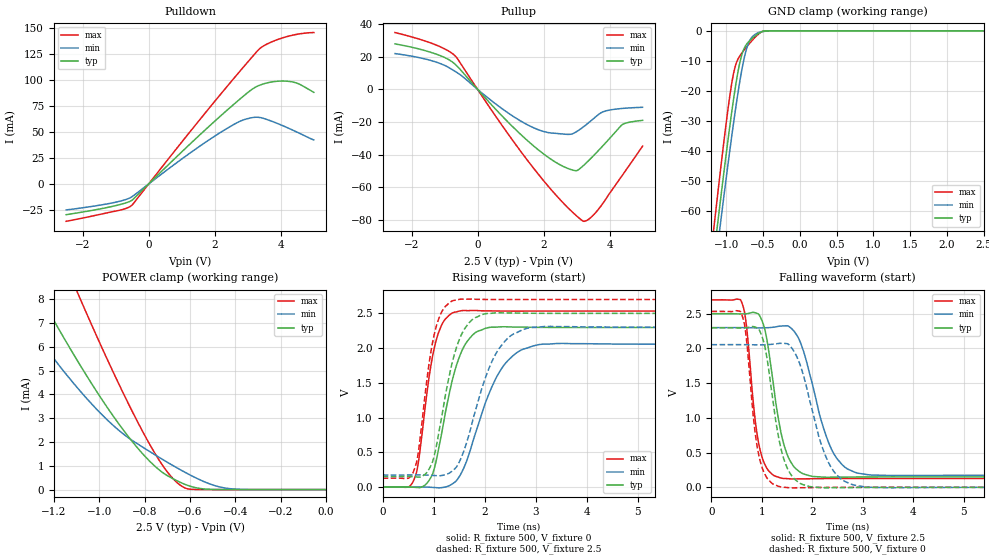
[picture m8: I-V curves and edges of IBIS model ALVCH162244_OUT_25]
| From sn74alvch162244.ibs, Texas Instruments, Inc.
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[Model]   ALVCH162244_OUT_25
Model_type  3-state
Enable   Active-Low
Vref =   0
Rref =   500
Cref =   30p
Vmeas =   1.25
| variable   typ   min   max
C_comp   7.01pF   5.81pF   8.07pF
| C_pullup   5.45pF   4.15pF   8.21pF
| C_pulldown   4.49pF   3.97pF   5.46pF
| C_tri-state   7.01pF   5.81pF   8.07pF
[Temperature Range]   40   100   -40
| Ambient temperature   25   85   -40
[Voltage range]   2.5   2.3   2.7
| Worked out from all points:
|   slope of the pulldown table from 0 to 0.375 V, typ, clamps not added: 32.2 ohm
|   slope of the pullup table from 0 to 0.375 V, typ, clamps not added: 44.6 ohm
|   GND clamp passes 1 mA (typ) near -0.57 V on its own axis
|   POWER clamp passes 1 mA (typ) near -0.76 V on its own axis
|   rising waveform, R_fixture 500, V_fixture 0: 20-80 % time 414ps typ, 616ps min, 291ps max; typ from 0 V to 2.3 V
|   falling waveform, R_fixture 500, V_fixture 2.5: 20-80 % time 313ps typ, 488ps min, 220ps max; typ from 2.5 V to 0.151 V
|   rising waveform, R_fixture 500, V_fixture 2.5: 20-80 % time 396ps typ, 559ps min, 284ps max; typ from 0.151 V to 2.5 V
|   falling waveform, R_fixture 500, V_fixture 0: 20-80 % time 307ps typ, 476ps min, 218ps max; typ from 2.3 V to 0 V
[GND Clamp]
| ALVCH162244_OUT_25
|   Voltage   I(typ)   I(min)   I(max)
-2.5V     -368.1mA   -367.2mA   -371.3mA
-1.175V   -76.67mA   -83.94mA   -67.56mA
-1.12V    -65.28mA   -72.86mA   -55.65mA
-1.075V   -56.11mA   -63.91mA   -46.11mA
-960mV    -33.67mA   -41.79mA   -23.46mA
-880mV    -19.7mA    -27.44mA   -12.2mA
-805mV    -9.656mA   -15.54mA   -8.049mA
-730mV    -4.751mA   -6.651mA   -5.626mA
-670mV    -3.059mA   -2.851mA   -3.862mA
-590mV    -1.419mA   -939uA     -1.764mA
-460mV    -11.33uA   -126uA     -6.688uA
2.5V      83.81pA    43.81nA    39.19pA
[POWER Clamp]
| ALVCH162244_OUT_25
|   Voltage   I(typ)   I(min)   I(max)
-2.5V     32.96mA    25.76mA    44.33mA
-1.415V   10.88mA    8.346mA    15.71mA
-1.39V    10.43mA    7.998mA    15.1mA
-1.265V   8.212mA    6.323mA    12.13mA
-1.095V   5.397mA    4.263mA    8.259mA
-1.075V   5.085mA    4.041mA    7.82mA
-945mV    3.18mA     2.753mA    5.07mA
-835mV    1.794mA    1.945mA    2.921mA
-725mV    748.5uA    1.292mA    1.078mA
-645mV    315uA      848.1uA    201uA
-430mV    586.9nA    45uA       19.76nA
-31.15fV  83.81pA    322.9pA    46.7pA
[Pulldown]
| ALVCH162244_OUT_25
|   Voltage   I(typ)   I(min)   I(max)
-2.5V     -29.57mA   -25mA      -35.92mA
-1.11V    -21.64mA   -18.3mA    -26.79mA
-720mV    -18.47mA   -15.27mA   -23.9mA
-510mV    -15.74mA   -12.3mA    -20.47mA
1.71V     51.84mA    39.79mA    68.05mA
2.535V    75.28mA    56.31mA    99.7mA
2.96V     86.7mA     62.36mA    115.6mA
3.205V    92.39mA    63.96mA    124.6mA
3.41V     95.38mA    63.53mA    131.1mA
4.02V     98.8mA     56.47mA    139.9mA
4.49V     96.76mA    49.79mA    143.7mA
5V        87.96mA    42.25mA    145.4mA
[Pullup]
| ALVCH162244_OUT_25
|   Voltage   I(typ)   I(min)   I(max)
-2.5V     27.76mA    21.84mA    34.68mA
-1.295V   21.81mA    16.89mA    27.4mA
-680mV    15.33mA    10.96mA    20.45mA
795mV     -17.39mA   -12.61mA   -23.59mA
1.72V     -35mA      -23.72mA   -48.83mA
2.725V    -48.31mA   -27.56mA   -72.15mA
2.995V    -49.8mA    -25.98mA   -77.31mA
3.195V    -46.88mA   -23.17mA   -80.61mA
3.595V    -38.91mA   -16.57mA   -75.04mA
3.855V    -33.31mA   -13.41mA   -68.1mA
4.37V     -21.83mA   -11.74mA   -53.08mA
5V        -19mA      -11.01mA   -34.76mA
[Ramp]
| ALVCH162244_OUT_25
| variable   typ   min   max
dV/dt_r   1.39/4.27E-10   1.25/6.48E-10   1.53/3.02E-10
dV/dt_f   1.42/3.31E-10   1.29/5.15E-10   1.55/2.30E-10
R_load = 500
[Rising Waveform]
| ALVCH162244_OUT_25
R_fixture =   500
C_fixture =   0
L_fixture =   0
V_fixture =   0
V_fixture_min = 0
V_fixture_max = 0
|   Time   V(typ)   V(min)   V(max)
0s        249.4uV    275uV      221.5uV
620ps     -2.589mV   2.187mV    116.2mV
710ps     -6.682mV   2.508mV    398.7mV
940ps     131.6mV    -2.695mV   1.72V
1.185ns   882.8mV    -4.875mV   2.372V
1.565ns   1.979V     233.7mV    2.541V
1.84ns    2.233V     818.6mV    2.541V
2.315ns   2.307V     1.686V     2.534V
3.155ns   2.299V     2.059V     2.533V
40ns      2.297V     2.055V     2.533V
[Falling Waveform]
| ALVCH162244_OUT_25
R_fixture =   500
C_fixture =   0
L_fixture =   0
V_fixture =   2.5
V_fixture_min = 2.3
V_fixture_max = 2.7
|   Time   V(typ)   V(min)   V(max)
0s        2.5V       2.3V       2.7V
620ps     2.497V     2.3V       2.625V
690ps     2.499V     2.299V     2.354V
960ps     2.466V     2.296V     553.9mV
1.095ns   2.147V     2.298V     279.6mV
1.435ns   620.9mV    2.325V     127mV
1.765ns   215.7mV    2.085V     122.4mV
2.435ns   146.8mV    474.3mV    126.6mV
3.165ns   149.6mV    177.1mV    127.2mV
40ns      150.8mV    173.8mV    127mV
[Rising Waveform]
| ALVCH162244_OUT_25
R_fixture =   500
C_fixture =   0
L_fixture =   0
V_fixture =   2.5
V_fixture_min = 2.3
V_fixture_max = 2.7
|   Time   V(typ)   V(min)   V(max)
0s        151mV      174.1mV    127.3mV
610ps     148.1mV    175.6mV    232.1mV
705ps     143.9mV    175.7mV    528.4mV
920ps     272.3mV    170.5mV    1.826V
1.165ns   1.039V     167.7mV    2.53V
1.355ns   1.764V     225.7mV    2.676V
1.535ns   2.178V     412.9mV    2.704V
2.255ns   2.509V     1.962V     2.7V
3.16ns    2.501V     2.311V     2.7V
40ns      2.5V       2.3V       2.7V
[Falling Waveform]
| ALVCH162244_OUT_25
R_fixture =   500
C_fixture =   0
L_fixture =   0
V_fixture =   0
V_fixture_min = 0
V_fixture_max = 0
|   Time   V(typ)   V(min)   V(max)
0s        2.297V     2.054V     2.533V
610ps     2.295V     2.055V     2.473V
685ps     2.297V     2.054V     2.194V
945ps     2.271V     2.052V     444mV
1.075ns   1.971V     2.054V     167.1mV
1.42ns    444.7mV    2.073V     375.5uV
1.73ns    71.1mV     1.821V     -5.64mV
2.375ns   -5.73mV    285.6mV    -923.1uV
3.11ns    -1.852mV   1.326mV    146.3uV
40ns      4.498nV    4.312nV    2.54nV
